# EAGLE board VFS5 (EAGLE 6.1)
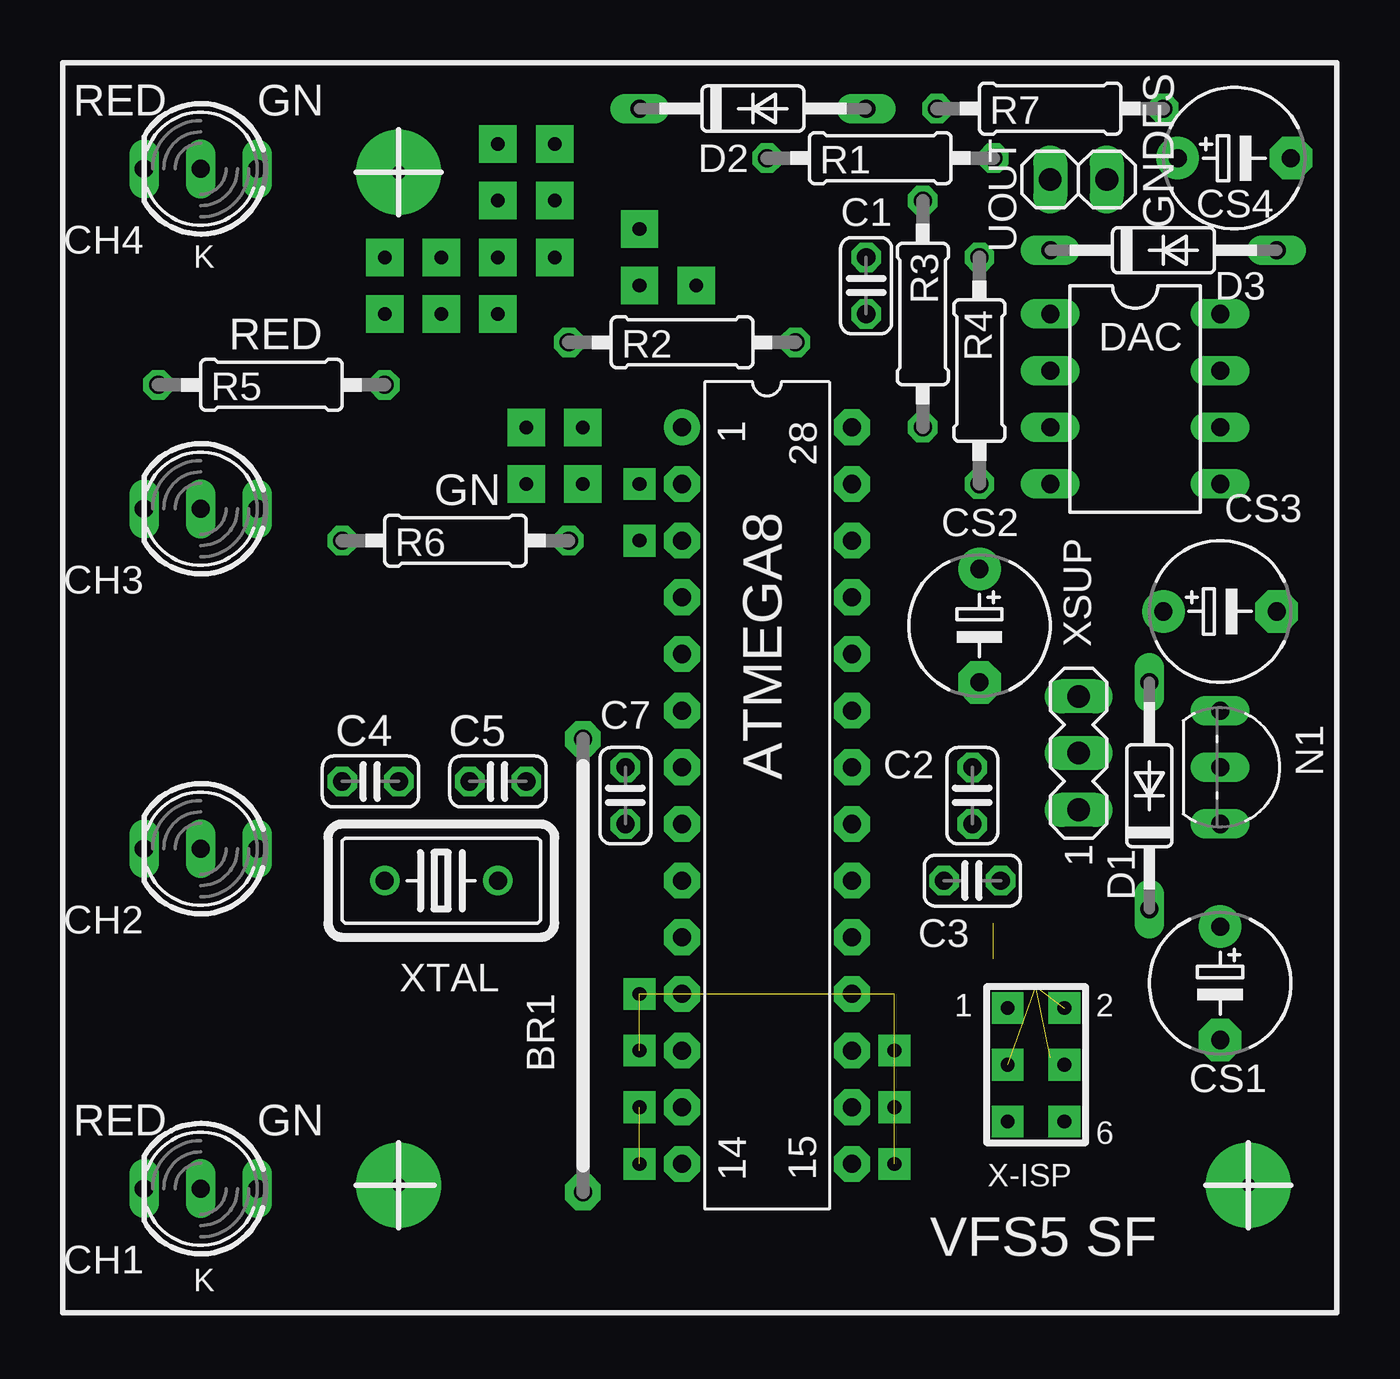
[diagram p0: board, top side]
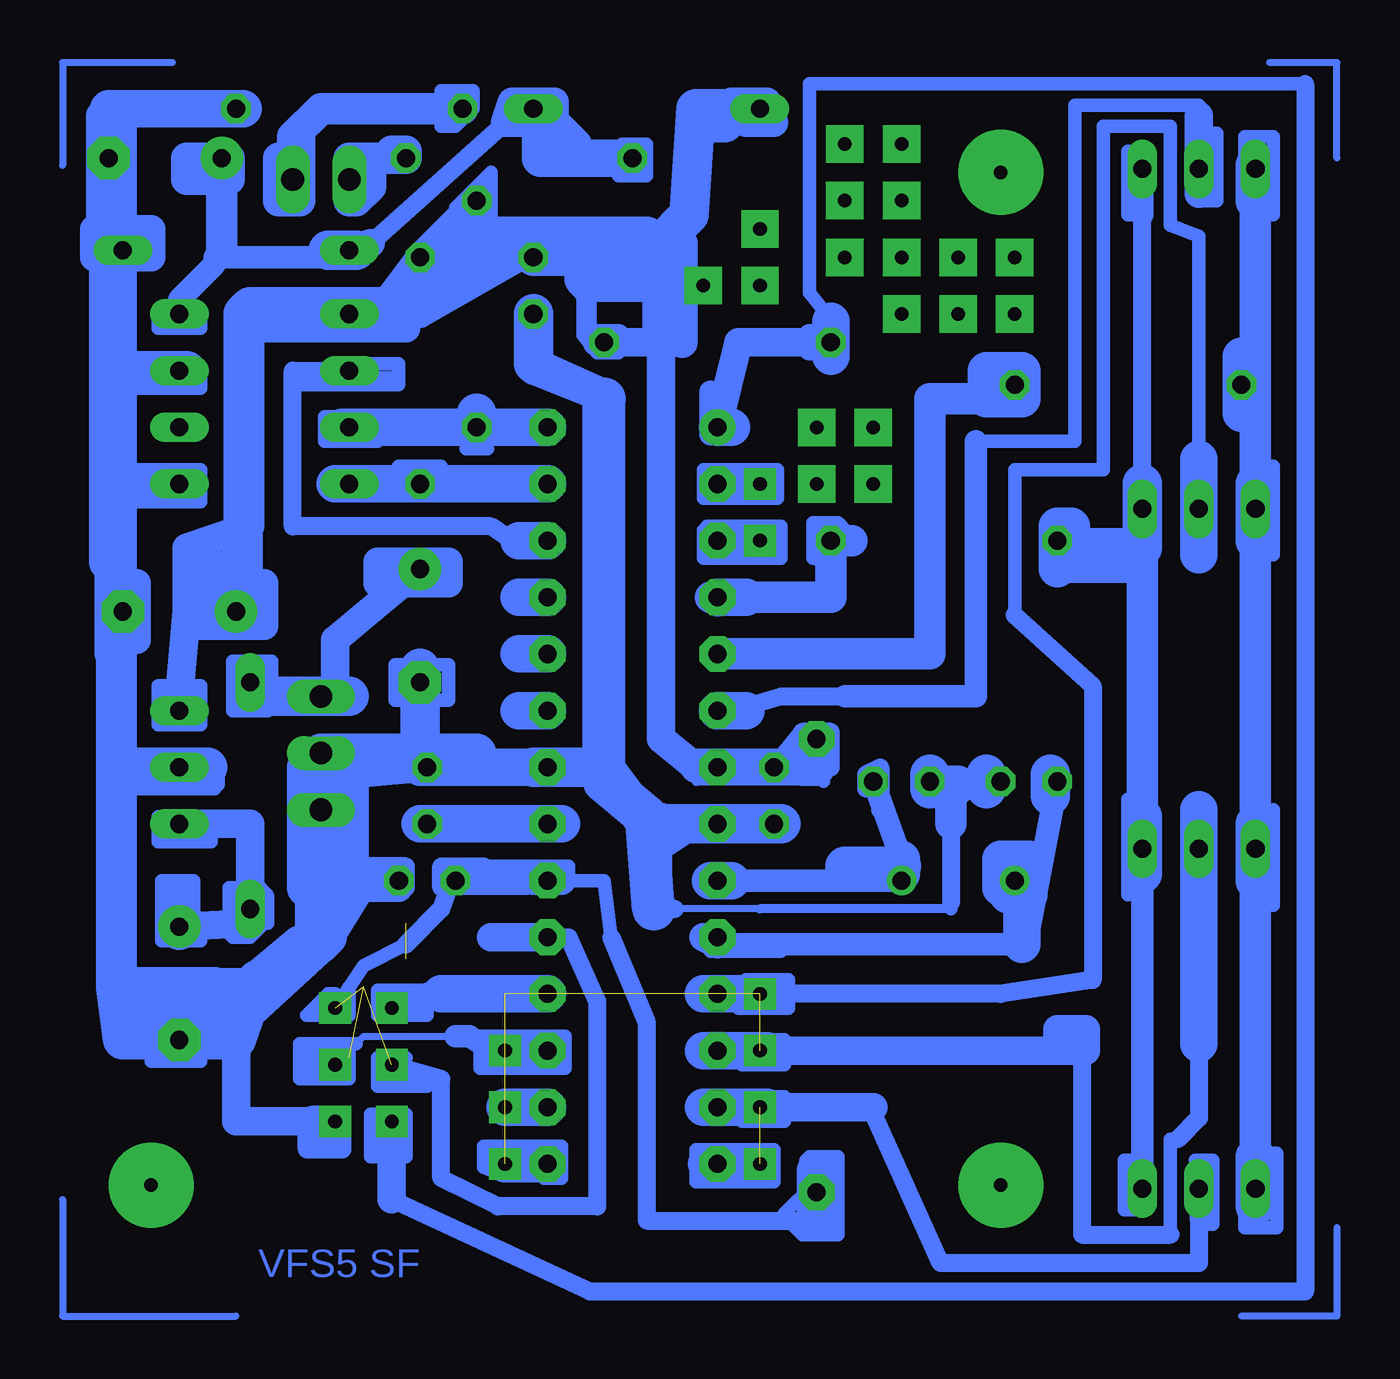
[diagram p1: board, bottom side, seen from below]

No outline drawn. Coordinates in mm, seen from the top.
Copper layers 16: Bottom 0.035mm
Design rules: minimum track width 10mil, minimum drill 24mil, track to track 8mil, track to pad 8mil, pad to pad 8mil, via to via 8mil, smd to smd 8mil, copper to edge 40mil, drill to drill 8mil, minimum pad ring 10mil, minimum via ring 8mil, stop-mask expansion 4mil, vias tented up to drill 0mil, thermal gap 10mil

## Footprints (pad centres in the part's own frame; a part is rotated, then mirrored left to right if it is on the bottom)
DIL28-3 = drill 0.813 pad 1.6: 1 -16.51,-3.81 | drill 0.813 pad 1.6 octagon: 2 -13.97,-3.81; 3 -11.43,-3.81; 4 -8.89,-3.81; 5 -6.35,-3.81; 6 -3.81,-3.81; 7 -1.27,-3.81; 8 1.27,-3.81; 9 3.81,-3.81; 10 6.35,-3.81; 11 8.89,-3.81; 12 11.43,-3.81; 13 13.97,-3.81; 14 16.51,-3.81; 15 16.51,3.81; 16 13.97,3.81; 17 11.43,3.81; 18 8.89,3.81; 19 6.35,3.81; 20 3.81,3.81; 21 1.27,3.81; 22 -1.27,3.81; 23 -3.81,3.81; 24 -6.35,3.81; 25 -8.89,3.81; 26 -11.43,3.81; 27 -13.97,3.81; 28 -16.51,3.81
20 = drill 0.813 pad 1.6 octagon: 1 -10.16,0; 2 10.16,0
C025-024X044 = drill 0.813 octagon: 1 -1.27,0; 2 1.27,0
DUOLED-A-5MM = drill 0.813 long: A 0,0; CR 2.54,0; CX -2.54,0
E5-6 = drill 0.813 pad 1.905: + -2.54,0 | drill 0.813 pad 1.905 octagon: - 2.54,0
DO35-10 = drill 0.813 long: A 5.08,0; C -5.08,0
DIL08 = drill 0.813 long: 1 -3.81,-3.81; 2 -1.27,-3.81; 3 1.27,-3.81; 4 3.81,-3.81; 5 3.81,3.81; 6 1.27,3.81; 7 -1.27,3.81; 8 -3.81,3.81
TO92-CEB = drill 0.813 long: B 2.54,0; C -2.54,0; E 0,0
0207/10 = drill 0.813 octagon: 1 -5.08,0; 2 5.08,0
1X02 = drill 1.016 long: 1 -1.27,0; 2 1.27,0
MA03-1 = drill 1.016 long: 1 -2.54,0; 2 0,0; 3 2.54,0
HC18U-V = drill 0.813: 1 -2.54,0; 2 2.54,0

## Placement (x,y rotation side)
ATMEGA8  ATmega8  [DIL28-3]  101.6,59.69 270 top
BR1  [20]  93.34,52.07 90 top
C1  [C025-024X044]  106.05,82.55 90 top
C2  [C025-024X044]  110.81,59.69 90 top
C3  [C025-024X044]  110.81,55.88 180 top
C4  [C025-024X044]  83.82,60.33 180 top
C5  [C025-024X044]  89.53,60.33 180 top
C7  [C025-024X044]  95.25,59.69 90 top
CH1  [DUOLED-A-5MM]  76.2,42.07 180 top
CH2  [DUOLED-A-5MM]  76.2,57.31 180 top
CH3  [DUOLED-A-5MM]  76.2,72.55 180 top
CH4  [DUOLED-A-5MM]  76.2,87.79 180 top
CS1  [E5-6]  121.92,51.28 270 top
CS2  [E5-6]  111.12,67.31 270 top
CS3  [E5-6]  121.92,67.94 0 top
CS4  [E5-6]  122.56,88.27 0 top
D1  [DO35-10]  118.75,59.69 90 top
D2  [DO35-10]  100.97,90.49 0 top
D3  [DO35-10]  119.38,84.14 0 top
DAC  [DIL08]  118.11,77.47 270 top
N1  [TO92-CEB]  121.92,60.96 270 top
R1  [0207/10]  106.68,88.27 0 top
R2  [0207/10]  97.79,80.01 0 top
R3  [0207/10]  108.58,81.28 90 top
R4  [0207/10]  111.12,78.74 90 top
R5  [0207/10]  79.38,78.11 180 top
R6  [0207/10]  87.63,71.12 180 top
R7  [0207/10]  114.3,90.49 0 top
UOUT  [1X02]  115.57,87.31 180 top
XSUP  [MA03-1]  115.57,61.59 90 top
XTAL  [HC18U-V]  87,55.88 0 top

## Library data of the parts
ATMEGA8 = PIC
BR1 = jumper
C1-C5 C7 CS1-CS4 R1-R7 = rcl
CH1-CH4 = led
D1-D3 = diode
DAC = ic-package
N1 = transistor-neu-to92
UOUT = pinhead-1
XSUP = Sigi-Lib
XTAL = crystal

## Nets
S$9: CS2.-
S$12: CS2.+
S$16: C1.2 CS3.+ DAC.1 N1.C R3.2 R4.2
S$18: CS1.+ D1.C
S$27: DAC.5 DAC.7 N1.E
S$37: ATMEGA8.17
S$38: C5.1
S$42: C4.2
S$43: ATMEGA8.18
S$45: C4.1
S$46: XTAL.2
S$50: CS4.+
S$55: ATMEGA8.6
S$60: R6.2
S$71: ATMEGA8.4
S$73: ATMEGA8.3
S$76: CH3.A
S$77: XSUP.2
S$86: DAC.8
S$88: BR1.1
S$91: R1.2
S$115: R7.1

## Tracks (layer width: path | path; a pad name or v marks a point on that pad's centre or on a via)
S$1
  Bottom 1.422: 114.62,61.28 111.12,61.28
S$2
  Bottom 1.676: 85.09,55.88 84.45,55.88
S$3
  Bottom 1.676: 105.41,76.2 108.58,76.2 114.62,76.2
  Bottom 1.778: 108.58,76.2 108.58,76.83
S$4
  Bottom 1.676: 105.41,73.66 114.94,73.66
S$5
  Bottom 1.422: 93.03,71.12 91.76,71.12
S$6
  Bottom 1.676: 105.41,68.58 106.68,68.58
S$7
  Bottom 1.676: 105.41,66.04 106.68,66.04
S$8
  Bottom 1.676: 105.41,63.5 106.68,63.5
S$9
  Bottom 1.27: 111.12,61.59 111.12,60.96
  Bottom 1.676: 106.36,60.96 111.12,60.96
  Bottom 1.778: 111.12,61.59 CS2.- 111.12,65.41
S$10
  Bottom 1.676: 104.78,58.42 107.63,58.42 111.12,58.42
S$11
  Bottom 1.778: 106.05,81.28 106.05,79.06
S$12
  Bottom 1.27: CS2.+ 114.94,66.67 114.94,64.14 | 114.3,64.14 114.94,64.14 | 114.94,64.14 118.75,64.14 | 118.75,64.77 118.75,65.41
  Bottom 1.778: 114.3,64.14 118.75,64.14 118.75,64.77
S$13  (via drill 0.61 pad 3.81)
  other vias: 85.09,42.23
S$14
  Bottom 1.422: 99.38,84.45 99.38,80.01
S$15
  Bottom 1.778: 100.97,84.77 109.22,84.77
S$16
  Bottom 1.27: 108.58,83.19 R3.2 R4.2 | 121.92,64.14 121.6,67.94 | 121.6,67.94 121.6,70.8 118.75,71.75 118.75,80.64 116.2,81.28 DAC.1 113.03,81.28 | 121.6,67.94 CS3.+ 119.38,69.22 | 113.03,81.28 111.12,81.28 | 111.12,81.28 106.68,83.82 C1.2 | R4.2 111.12,81.28 | R4.2 113.03,81.28 | R4.2 107.31,83.82 | 119.38,69.22 119.38,71.12 | 119.38,69.22 118.11,69.22 118.11,67.31 121.28,67.31
  Bottom 1.676: C1.2 103.5,83.82
  Bottom 1.778: N1.C 121.92,64.14
S$17  (via drill 0.61 pad 3.81)
  other vias: 123.19,42.23
S$18
  Bottom 1.27: 122.56,58.42 118.75,58.42 D1.C 118.75,53.98 CS1.+
S$19  (via drill 0.61 pad 3.81)
  other vias: 85.09,87.63
S$20
  Bottom 0.305: 95.89,54.61 99.69,54.61 | 100.33,54.61 100.65,54.61
  Bottom 0.406: 87.31,54.61 95.89,54.61
  Bottom 0.61: 87.31,54.93 87.31,54.61
  Bottom 0.813: 87.95,60.01 87.31,59.37 | 87.31,58.42 87.31,54.93 | 99.69,54.61 100.33,54.61
  Bottom 1.422: 87.31,59.37 87.31,58.42
S$21
  Bottom 1.422: 73.66,87.63 73.66,86.36 73.66,73.66 | 73.66,71.12 73.66,58.42 | 73.66,55.88 73.66,43.5
  Bottom 1.778: 73.66,58.42 73.66,55.88 | 73.66,43.5 73.66,41.27 | 73.66,73.66 73.66,71.12 | 73.66,87.95 73.66,86.36
S$22
  Bottom 0.813: 107.31,89.85 113.35,84.45
  Bottom 1.27: 113.35,84.45 114.3,84.14 | 107.31,89.85 105.09,89.85 105.09,90.81 107,90.81 107.31,89.85
  Bottom 1.778: 113.98,84.14 114.3,84.14 115.25,84.14
S$23
  Bottom 1.778: 108.9,83.5 110.17,82.23 111.76,82.23 112.39,81.6 118.43,81.6 118.43,80.96
S$24  (via drill 0.61 pad 1.42, 0.61 pad 1.68)  (1 unrouted)
  other vias: 95.89,45.72 95.89,43.18 84.45,81.28 87,81.28 89.53,81.28 89.53,83.82 87,83.82 84.45,83.82 89.53,86.36 89.53,88.9 95.89,71.12 95.89,73.66 93.34,73.66 93.34,76.2 95.89,82.55 98.42,82.55 95.89,85.09 92.08,88.9 92.08,86.36 92.08,83.82 90.81,76.2 90.81,73.66
S$25
  Bottom 1.27: 123.19,85.09 125.41,85.09 125.73,85.09 125.73,83.82 123.19,83.82 123.19,85.09
  Bottom 1.422: 125.41,90.17 125.41,85.09
S$26  (1 unrouted)
S$27  (via drill 0.61 pad 1.42)
  Bottom 1.27: v114.94,45.09 119.38,45.09 119.38,48.74 | 114.62,55.56 113.98,55.56 112.08,55.56 112.08,55.88 113.35,55.88 | 118.43,51.44 119.38,50.8 119.38,50.16 124.46,50.16 124.46,60.96 | 124.46,90.49 124.46,78.74 | 124.46,78.74 124.46,73.66 | 124.46,73.66 124.46,60.96 | N1.E 124.46,60.96 | 123.83,73.66 124.46,73.66 | DAC.7 123.83,78.74 124.46,78.74
  Bottom 1.422: v114.94,45.09 115.89,45.09
  Bottom 1.676: 113.98,55.56 115.57,53.02 115.25,53.34 | 115.25,60.33 115.25,53.34 | 115.25,53.34 116.52,53.02 118.43,51.44 | 115.25,53.34 119.06,49.85 119.38,48.74
  Bottom 1.778: 124.78,66.04 124.78,51.12 124.46,48.74 119.38,48.74 118.43,51.44 | 120.65,60.96 124.46,60.96 | 121.6,78.74 123.83,78.74 | 121.6,73.66 DAC.5 123.83,73.66
S$28
  Bottom 1.676: 125.09,90.49 123.51,90.49
S$29
  Bottom 1.676: 119.06,90.49 124.14,90.49
S$30
  Bottom 0.61: 97.47,89.85 96.52,89.85 97.16,90.01
  Bottom 0.813: 97.16,90.01 97.47,89.85
  Bottom 1.27: 97.16,90.17 97.16,90.81 95.57,90.81 95.25,89.85 96.52,89.85
S$31
  Bottom 1.27: 111.76,80.64 118.11,80.64
S$32
  Bottom 1.27: 125.09,69.85 125.09,66.04
S$33
  Bottom 0.813: 76.2,41.91 76.2,40.64 | 76.2,40.64 76.2,38.73 87.79,38.73 90.81,45.4 | 76.2,40.64 76.2,43.18
S$34
  Bottom 1.27: 123.83,66.67 123.83,69.22
S$35
  Bottom 1.016: 84.14,53.02 97.79,53.02
  Bottom 1.27: 98.42,53.34 97.79,53.02
  Bottom 1.676: 83.82,55.88 84.14,55.88 84.14,53.02
S$36
  Bottom 1.27: 120.65,68.58 120.65,70.48
S$37
  Bottom 1.676: ATMEGA8.17 107.63,48.26
S$38
  Bottom 1.016: C5.1 89.53,56.83
  Bottom 1.676: 89.53,56.2 89.53,56.52 89.53,56.83
  Bottom 1.778: 89.53,56.52 92.08,56.52
S$39
  Bottom 1.676: 85.09,55.56 85.09,56.83
S$40
  Bottom 1.676: 84.77,55.24 83.82,55.24 83.82,56.83 85.09,56.83
S$41  (via drill 0.61 pad 1.42)  (3 unrouted)
  Bottom 0.61: v114.94,50.16 113.67,52.07 111.76,53.02
  Bottom 0.813: 105.41,53.34 104.46,53.34 103.19,50.48 103.19,41.27 107.63,41.27 110.17,42.55 110.17,46.99 v112.39,47.62 | 109.86,55.56 110.17,54.61 111.76,53.02
  Bottom 1.27: 105.41,53.34 107.95,53.34
S$42
  Bottom 1.016: C4.2 83.82,53.66
S$43  (via drill 0.61 pad 1.42)
  Bottom 1.016: v112.39,50.16 110.81,50.8 110.17,50.8
  Bottom 1.676: ATMEGA8.18 110.17,50.8
S$44
  Bottom 1.422: 97.79,68.42 98.11,68.58
S$45
  Bottom 1.016: C4.1 88.27,60.33
S$46
  Bottom 1.016: 98.42,55.88 98.11,55.88 90.81,55.88 90.49,55.88 XTAL.2
  Bottom 1.676: 98.11,55.88 97.16,55.88
S$47  (via drill 0.61 pad 1.42)
  Bottom 0.61: 71.44,91.6 93.66,91.6 93.66,82.23 92.39,80.64 92.71,80.96
  Bottom 0.813: 112.39,41.59 103.5,37.47 71.44,37.47 71.44,91.6
  Bottom 1.27: 112.39,41.59 v112.39,45.09
  Bottom 1.676: 92.71,80.96 92.71,79.38
S$48
  Bottom 1.27: 95.89,45.72 90.81,45.72
  Bottom 1.676: 98.42,45.72 95.89,45.72 95.57,45.72
S$49
  Bottom 1.27: 95.89,48.26 81.28,48.26 81.28,49.21 82.55,49.21 82.55,48.58
  Bottom 1.676: 98.42,48.26 95.89,48.26 95.57,48.26
S$50
  Bottom 1.422: CS4.+ 120.02,84.14
S$51
  Bottom 1.778: 118.75,81.6 119.06,81.28 119.06,68.9
S$52
  Bottom 1.27: 92.71,80.01 96.84,80.01 97.79,76.2
  Bottom 1.676: 97.79,76.2 97.16,76.2
S$53
  Bottom 1.676: 100.65,58.1 100.65,54.61
S$54
  Bottom 0.813: 85.72,60.01 85.41,60.64 85.72,60.64
  Bottom 1.778: 85.72,60.64 85.72,60.01
S$55
  Bottom 0.61: 86.2,75.56 81.76,75.56 81.76,90.65 76.2,90.65 76.2,90.17 76.2,87
  Bottom 0.813: 97.16,63.5 94.93,64.14 92.08,64.14 91.76,64.14
  Bottom 1.016: 92.08,64.14 86.2,64.14 86.2,75.56
  Bottom 1.27: 76.2,86.68 76.2,90.17
  Bottom 1.676: ATMEGA8.6 97.16,63.5 96.52,63.5
S$56
  Bottom 0.813: 90.49,60.96 91.12,60.64 91.12,60.01 90.49,60.96 | 90.49,60.96 90.49,59.05
S$57
  Bottom 1.422: 87,60.01 87.95,60.01
S$58
  Bottom 1.422: 87.63,59.69 87.95,60.33
S$59
  Bottom 1.422: 87,60.33 87.95,60.33
S$60
  Bottom 0.61: 78.74,43.34 79.53,43.34 79.53,41.12 78.9,41.12
  Bottom 0.813: 78.74,73.66 78.74,85.72
  Bottom 1.016: 78.74,56.2 78.74,43.34 78.74,41.59 | 78.74,88.27 78.74,85.72
  Bottom 1.27: R6.2 82.55,70.48 | 82.55,69.85 78.74,69.85
  Bottom 1.422: 78.74,58.74 78.74,69.85 78.74,70.8
  Bottom 1.676: 82.55,70.48 81.92,70.48 81.92,71.75 82.55,71.75 82.55,70.48 | 82.55,70.48 82.55,69.85
  Bottom 1.778: 78.74,58.74 78.74,56.2 | 78.74,73.66 78.74,70.8 81.28,70.8
S$61
  Bottom 1.676: 101.92,88.27 105.73,88.27 105.73,90.49
S$62
  Bottom 1.016: 98.11,75.88 98.11,77.79
S$63
  Bottom 1.016: 92.39,80.33 92.39,79.69 93.66,79.69 93.66,80.33 92.39,80.33
S$64
  Bottom 1.27: 109.86,70.17 113.03,70.17 113.03,69.22 109.86,69.22 109.86,70.17
S$65
  Bottom 1.676: 105.41,43.18 107.31,43.18
S$66
  Bottom 1.676: 107.31,45.72 105.41,45.72
S$67
  Bottom 0.813: 92.71,60.96 92.71,62.55 93.98,62.55 95.25,60.96
  Bottom 1.016: 98.74,60.96 98.42,60.64
  Bottom 1.27: 103.19,80.01 100.33,80.01 100.33,62.23 98.74,60.96
  Bottom 1.422: 94.3,60.96 95.25,60.96 98.74,60.96
  Bottom 1.676: 103.82,82.87 103.82,84.14 100.33,84.45 100.33,80.01
  Bottom 1.778: 97.16,90.49 98.74,90.49 99.06,85.72 100.33,84.45
S$68
  Bottom 0.813: 90.49,55.88 89.22,55.88 89.53,56.83
S$69
  Bottom 1.016: 101.28,80.01 103.19,80.01 103.19,80.33 102.23,80.33
S$70
  Bottom 1.422: 104.14,88.9 105.41,90.17
S$71
  Bottom 1.422: 96.52,68.58 92.71,68.58 92.71,71.12
  Bottom 1.676: 96.52,68.58 ATMEGA8.4
S$72
  Bottom 0.813: 76.2,48.58 76.2,45.24 77.15,44.29
  Bottom 1.676: 76.2,48.58 76.2,59.05
S$73
  Bottom 1.422: ATMEGA8.3 96.52,71.12
S$74
  Bottom 1.676: 74.3,79.38 74.3,76.83
S$75
  Bottom 1.422: 114.94,60.64 111.44,60.96
S$76
  Bottom 0.61: 77.47,89.69 77.47,85.25 76.2,84.77 76.2,74.77 CH3.A
  Bottom 1.676: 76.2,74.77 76.2,70.48
S$77
  Bottom 1.778: XSUP.2 108.58,61.59
S$78
  Bottom 1.676: 118.43,51.12 122.87,51.12
  Bottom 1.778: 120.33,51.12 122.87,51.12 123.83,51.12
S$79
  Bottom 0.305: 70.01,88.27 70.01,92.55 73.03,92.55
S$80
  Bottom 0.305: 122.24,92.55 127.16,92.55 127.16,87.95
S$81
  Bottom 0.305: 127.16,41.59 127.16,36.35 119.38,36.35
S$82
  Bottom 0.305: 70.01,40.32 70.01,36.35 74.3,36.35
S$83
  Bottom 0.61: 84.45,67.79 84.45,74.3 80.49,74.3 80.49,89.69 77.63,89.69
  Bottom 0.813: 96.2,50.8 85.09,50.8 80.96,51.44 80.96,64.61 84.45,67.79
S$84
  Bottom 1.422: 97.47,66.04 88.27,66.04 88.27,77.47 84.45,77.47
  Bottom 1.676: 84.45,78.74 84.45,77.47 | 84.45,77.47 84.14,77.47 84.14,78.74 85.72,78.74 85.72,77.47 84.45,77.47
S$85
  Bottom 1.676: 93.98,60.96 93.34,60.96
S$86
  Bottom 1.016: 115.57,83.82 120.33,83.82 120.33,83.5 121.92,81.92 DAC.8
S$87
  Bottom 1.016: 98.11,53.02 96.84,53.02
S$88
  Bottom 0.305: 109.86,55.24 109.54,55.88
  Bottom 0.61: 104.78,55.88 102.87,55.88 102.55,53.34
  Bottom 0.813: 102.55,53.34 100.97,49.53 100.97,40.64 93.34,40.64 BR1.1
  Bottom 1.016: 108.58,55.88 108.9,55.88 | 106.05,55.88 106.36,55.88
  Bottom 1.27: 109.86,55.88 109.54,55.88 108.58,55.88 106.36,55.88 | 104.78,55.88 106.05,55.88
  Bottom 1.778: 93.34,40.64 93.34,40.96 93.34,42.86
S$89
  Bottom 1.778: 125.09,83.19 125.09,70.17
S$90
  Bottom 1.422: 120.33,88.27 121.6,88.27 121.6,87.31 119.7,87.31 119.7,88.27
S$91
  Bottom 1.422: 113.35,87.63 113.35,87 113.98,86.36 114.3,86.36 114.3,88.27 R1.2 111.76,88.58 112.39,88.58
S$92  (via drill 0.61 pad 1.42)
  other vias: 114.94,47.62
S$93
  Bottom 1.778: 121.92,55.24 121.92,53.66
S$94
  Bottom 1.778: 82.87,60.64 82.87,59.69
S$95
  Bottom 1.778: 88.27,60.64 88.27,60.01
S$96
  Bottom 1.676: 98.42,50.8 95.57,50.8
S$97
  Bottom 0.61: 77.47,44.29 77.47,40.01
  Bottom 0.813: 81.44,48.42 81.44,40.01 77.47,40.01
S$98
  Bottom 1.422: 98.42,43.18 95.89,43.18
S$99  (via drill 0.61 pad 1.42)  (5 unrouted)
  other vias: 95.89,50.8 95.89,48.26 107.31,43.18 107.31,45.72 107.31,48.26
S$100
  Bottom 0.813: 114.62,45.09 114.62,43.81 116.2,43.81 116.2,44.77
S$101
  Bottom 1.27: 102.87,77.47 106.05,78.74
  Bottom 1.676: 100.97,58.74 100.01,58.42
  Bottom 1.778: 106.05,60.96 102.87,60.96 100.97,58.42 100.01,58.42 94.93,58.42
  Bottom 1.93: 100.65,54.61 100.97,58.74 102.87,60.33 102.87,77.47
S$102
  Bottom 0.61: 111.44,50.8 113.03,50.8 113.03,49.85 110.81,49.85 110.81,50.16
S$103
  Bottom 1.676: 115.89,55.56 115.89,53.98
S$104
  Bottom 0.61: 114.3,51.12 114.3,49.85 116.2,49.85 115.25,50.8 114.94,50.8
S$105
  Bottom 0.305: 114.62,47.94 113.98,48.58 113.67,48.9 109.54,48.9
  Bottom 0.61: 114.3,48.58 114.3,46.99 116.52,46.99 116.52,48.58 113.98,48.58
  Bottom 1.016: 107.95,48.26 108.9,48.9 109.54,48.9
S$106
  Bottom 1.27: 97.47,73.66 97.79,73.66
  Bottom 1.676: 97.79,73.66 96.84,73.66
S$107
  Bottom 0.813: 115.89,44.45 114.94,44.45
S$108
  Bottom 1.778: 97.47,89.85 98.11,89.85
S$109
  Bottom 1.778: 116.2,60.96 116.2,55.56
S$110
  Bottom 0.61: 115.89,48.26 115.89,47.31 116.2,48.26
S$111
  Bottom 0.61: 111.76,47.94 113.03,47.94 113.03,46.67 110.81,46.67 110.81,46.99 111.76,46.99
S$112
  Bottom 0.61: 111.76,45.4 111.76,43.5 113.35,43.5 113.35,45.4 111.76,45.4
S$113
  Bottom 0.813: 111.76,55.56 111.76,56.52 114.3,56.52 114.94,56.52
  Bottom 1.778: 114.3,60.33 114.3,56.52
S$114
  Bottom 0.61: 109.54,86.04 107.95,87.63 107.95,85.41
S$115
  Bottom 1.422: R7.1 115.57,90.49 116.84,89.22 116.84,88.27 | 116.84,88.27 116.84,87 | 116.84,88.27 117.47,88.27 117.47,86.36 116.52,86.36 116.52,89.22
S$116
  Bottom 0.61: 76.04,40.48 75.56,40.48 75.56,43.34 76.36,43.34
S$117
  Bottom 0.61: 78.74,88.58 79.38,88.58 79.38,85.72 79.06,85.72
S$118
  Bottom 0.61: 113.98,79.06 112.08,79.06 112.08,78.11 116.52,78.11
S$119
  Bottom 0.61: 112.39,78.42 113.67,78.42 114.94,78.74
  Bottom 0.813: 106.68,71.12 107,71.12 107.95,71.75 116.84,71.75 116.84,78.74 114.94,78.74 114.3,78.74
  Bottom 1.676: 105.41,71.12 106.68,71.12
S$120
  Bottom 0.61: 103.5,80.01 103.5,80.33 103.5,82.55
  Bottom 1.016: 100.97,82.55 103.5,82.55 103.82,82.55
S$121
  Bottom 0.813: 103.19,83.19 100.97,83.19
S$122
  Bottom 0.61: 75.88,89.38 75.41,89.38 75.41,86.36 76.2,86.36
S$123
  Bottom 0.813: 104.14,82.55 103.82,82.23 100.97,82.23
S$124
  Bottom 0.61: 74.14,87.79 74.14,89.22 72.87,89.22 72.87,85.72 73.82,85.72
S$125
  Bottom 0.61: 73.03,74.45 72.87,74.45 72.87,70.48 73.03,70.48
S$126
  Bottom 0.61: 72.87,59.05 72.87,54.77
S$127
  Bottom 0.61: 79.38,59.53 79.38,55.24
S$128
  Bottom 0.61: 73.18,43.66 72.71,43.66 72.71,40.32 74.14,40.32 74.14,40.96
S$129
  Bottom 0.61: 96.52,51.44 94.61,51.44 94.61,50.16 96.84,50.16
S$130
  Bottom 0.61: 96.84,43.81 96.68,43.81 95.25,43.81 95.25,42.39 98.74,42.39 98.74,43.81 96.84,43.81
S$131
  Bottom 0.813: 99.38,57.78 100.33,57.15
S$132
  Bottom 0.406: 93.03,60.33 98.74,60.33
  Bottom 0.61: 93.03,60.33 94.3,61.28
S$133
  Bottom 0.406: 93.98,61.59 99.06,61.59
S$134
  Bottom 0.61: 102.87,78.11 105.73,79.38
S$135
  Bottom 0.61: 105.57,42.55 104.78,42.55 104.78,43.97 108.27,43.97 108.27,43.02 107.47,42.7
S$136
  Bottom 0.61: 108.43,48.9 104.62,48.9 104.62,47.47 108.43,47.47 108.43,48.42
S$137
  Bottom 0.61: 110.97,50.96 113.03,50.96
S$138
  Bottom 0.61: 110.17,74.45 112.08,74.45
S$139
  Bottom 0.61: 108.11,75.25 109.06,75.25
S$140
  Bottom 0.61: 102.23,79.53 103.19,79.53 103.82,80.33 103.82,82.39
S$141
  Bottom 0.61: 94.93,52.7 98.11,52.7
S$142
  Bottom 0.61: 104.46,56.2 104.46,56.52 108.27,56.52
  Bottom 0.813: 110.17,55.56 110.17,56.52 108.27,56.52
S$143
  Bottom 0.61: 102.08,88.9 100.97,88.9 100.97,87.47 102.23,87.47 102.23,88.11
S$144
  Bottom 0.61: 108.74,91.28 108.74,90.49 109.54,89.69 110.17,89.69 110.17,91.28 108.9,91.28
S$145
  Bottom 0.61: 123.98,74.3 120.97,74.3 120.97,72.87 123.83,72.87
S$146
  Bottom 0.61: 120.97,81.44 120.97,80.64 122.87,80.64 122.87,81.12
S$147
  Bottom 0.61: 120.97,78.58 120.97,77.95 123.83,77.95
S$148
  Bottom 0.61: 113.19,76.68 115.41,76.68 115.41,75.56 113.03,75.56
S$149
  Bottom 0.61: 110.97,65.72 110.97,65.56 109.86,65.56 109.86,63.98 112.24,63.98 112.24,65.56 111.76,65.56
S$150
  Bottom 0.61: 117.79,64.77 117.79,65.72 119.54,65.72 119.54,63.5 117.95,63.5
S$151
  Bottom 0.61: 120.97,64.45 120.97,62.87 122.87,62.87 122.87,64.61 120.97,64.61
S$152
  Bottom 0.61: 120.17,60.8 120.17,60.17 120.33,60.17 120.33,60.01 124.14,60.01
S$153
  Bottom 0.61: 120.33,58.74 122.87,58.74 122.87,57.63 120.49,57.63 120.49,58.1
S$154
  Bottom 0.61: 118.27,55.4 arc90 117.95,55.09 117.95,53.98 118.11,53.98 118.75,53.34 119.54,53.34 119.7,53.5 119.7,55.56 118.27,55.56
S$155
  Bottom 0.61: 120.97,53.98 120.97,53.18 122.71,53.18 122.71,55.88 121.28,55.88 121.28,54.45
S$156
  Bottom 0.61: 120.97,47.78 123.19,47.78
S$157
  Bottom 0.61: 98.42,74.3 95.09,74.3 95.09,73.03 98.42,73.03 98.42,74.3
S$158
  Bottom 0.61: 98.27,71.44 98.27,71.75 94.93,71.75 94.93,70.33 98.42,70.33 98.42,71.6
S$159
  Bottom 0.61: 92.08,71.6 92.39,71.91 93.5,71.91 93.5,70.33 93.34,70.33 93.19,70.17
S$160
  Bottom 0.61: 96.84,48.74 94.77,48.74 94.77,47.62 96.68,47.62
S$161
  Bottom 0.61: 96.52,46.2 94.77,46.2 94.77,45.09 96.68,45.09
S$162
  Bottom 0.61: 93.5,42.86 93.5,42.23 94.77,40.96 94.77,40.8 93.98,40.01 92.39,40.01 92.39,43.5 93.66,43.5 93.82,43.34

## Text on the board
Bottom: VFS5 SF
tPlace: VFS5 SF
tNames: GNDFS | RED | GN | K | RED | GN | C4 | C5 | 1 | 2 | 6 | RED | GN | X-ISP | K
